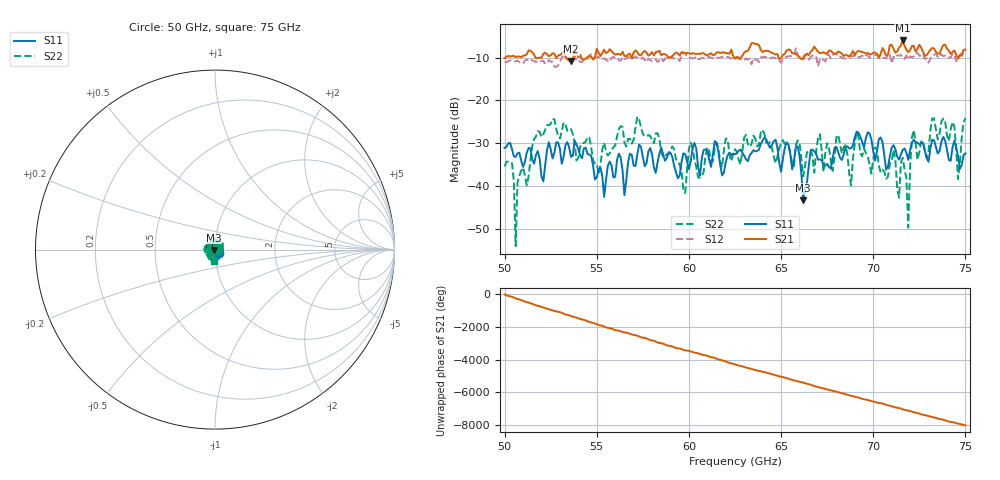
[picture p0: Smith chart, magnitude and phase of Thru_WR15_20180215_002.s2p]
# GHz S RI R 50
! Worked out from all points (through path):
!   251 points, 50 GHz to 75 GHz, reference 50 ohm
!   highest |S21| = -5.97 dB at 71.6 GHz (marker M1); lowest = -10.9 dB at 53.6 GHz (marker M2)
!   lowest |S11| = -43.4 dB at 66.2 GHz (marker M3), VSWR 1.01, Z = 49.3 - j0.141 ohm
!   |S11| at or under -10 dB: start of sweep to end of sweep
!   |S22| runs from -54.1 to -23.8 dB; largest |S21 - S12| = 0.78
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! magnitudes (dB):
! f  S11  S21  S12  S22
! 50 GHz  -31.1  -10.1  -11.0  -35.4
! 50.4 GHz  -31.4  -9.6  -10.8  -34.7
! 50.6 GHz  -33.2  -9.8  -10.9  -54.1
! 50.7 GHz  -32.4  -9.7  -10.7  -39.3
! 51.6 GHz  -34.8  -9.3  -10.8  -29.0
! 53.6 GHz  -33.2  -10.9  -10.6  -26.7
! 54.2 GHz  -33.5  -10.3  -11.1  -30.0
! 55.4 GHz  -42.6  -8.1  -10.2  -29.9
! 58.4 GHz  -32.4  -8.4  -10.6  -28.9
! 59.8 GHz  -32.6  -9.0  -8.9  -41.7
! 60.1 GHz  -34.2  -9.1  -10.0  -29.9
! 62.5 GHz  -32.6  -10.2  -9.8  -31.4
! 65.9 GHz  -30.8  -9.6  -9.3  -29.4
! 66.2 GHz  -43.4  -10.4  -9.8  -37.8
! 66.7 GHz  -31.5  -8.2  -9.5  -33.0
! 70.9 GHz  -33.1  -7.1  -9.3  -34.9
! 71.6 GHz  -31.6  -6.0  -10.1  -33.4
! 71.9 GHz  -33.9  -8.7  -10.4  -49.8
! 72.2 GHz  -29.2  -7.2  -9.7  -26.9
! 74.3 GHz  -31.0  -8.7  -9.1  -25.1
! 74.6 GHz  -33.1  -10.2  -10.3  -38.4
! 75 GHz  -32.4  -8.1  -9.4  -24.1
